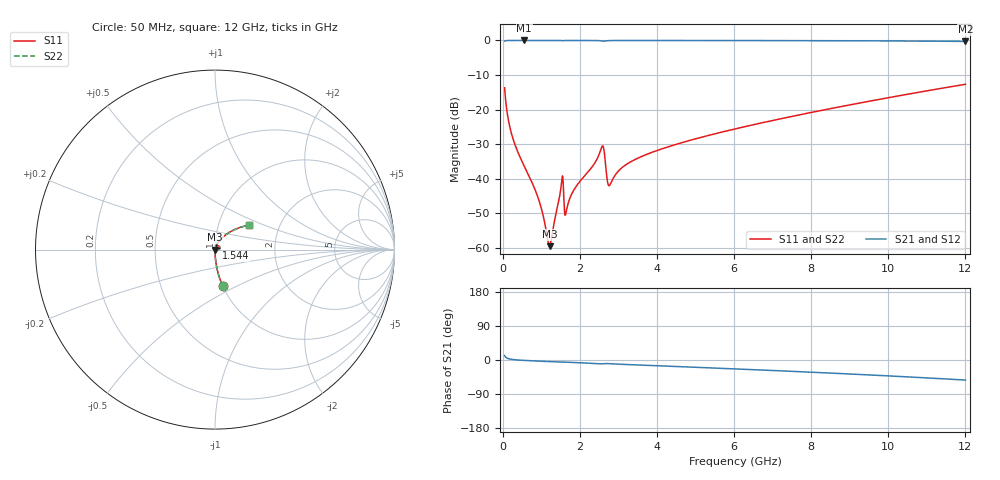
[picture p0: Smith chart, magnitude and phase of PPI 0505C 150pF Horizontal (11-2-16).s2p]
# MHz S MA R 50
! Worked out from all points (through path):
!   1601 points, 50 MHz to 12 GHz, reference 50 ohm
!   highest |S21| = -0.01 dB at 557.9 MHz (marker M1); lowest = -0.3 dB at 12 GHz (marker M2)
!   group delay of S21, straight-line fit = 12.3 ps
!   lowest |S11| = -59.5 dB at 1.215 GHz (marker M3), VSWR 1.00, Z = 50.1 - j0.00798 ohm
!   |S11| at or under -10 dB: start of sweep to end of sweep
!   |S22| runs from -59.5 to -12.7 dB; largest |S21 - S12| = 0
!   S11 on the Smith chart (normalised r, x): 50 MHz: 1.00, -0.42; 1.544 GHz: 1.02, +0.01; 12 GHz: 1.40, +0.40
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50  0.2069 -78.2  0.9781 11.8  0.9781 11.8  0.2069 -78.2
154.5625  0.06732 -86.3  0.9973 3.3  0.9973 3.3  0.06732 -86.3
236.7188  0.04311 -87.7  0.9985 1.7  0.9985 1.7  0.04311 -87.7
557.875  0.01524 -88.3  0.9991 -1.0  0.9991 -1.0  0.01524 -88.3
931.3125  0.005035 -82.5  0.999 -2.9  0.999 -2.9  0.005035 -82.5
1215.125  0.001054 -4.3  0.9989 -4.2  0.9989 -4.2  0.001054 -4.3
1274.875  0.001466 37.1  0.9988 -4.4  0.9988 -4.4  0.001466 37.1
1506.406  0.007098 62.6  0.9972 -5.6  0.9972 -5.6  0.007098 62.6
1543.75  0.01055 41.2  0.9927 -5.8  0.9927 -5.8  0.01055 41.2
1655.781  0.00349 53.9  0.9981 -5.9  0.9981 -5.9  0.00349 53.9
1805.156  0.006235 70.8  0.9985 -6.6  0.9985 -6.6  0.006235 70.8
2044.156  0.009735 73.7  0.9984 -7.6  0.9984 -7.6  0.009735 73.7
2566.969  0.02845 47.7  0.9844 -10.2  0.9844 -10.2  0.02845 47.7
2619.25  0.02754 17.4  0.9752 -9.7  0.9752 -9.7  0.02754 17.4
2716.344  0.009136 11.8  0.9913 -9.5  0.9913 -9.5  0.009136 11.8
2776.094  0.008046 42.2  0.9949 -9.9  0.9949 -9.9  0.008046 42.2
3186.875  0.01577 71.0  0.9977 -11.8  0.9977 -11.8  0.01577 71.0
4038.312  0.02594 70.5  0.9975 -15.3  0.9975 -15.3  0.02594 70.5
6025  0.05239 64.0  0.9959 -23.5  0.9959 -23.5  0.05239 64.0
8019.156  0.09113 55.9  0.9924 -32.3  0.9924 -32.3  0.09113 55.9
10013.31  0.1487 46.6  0.9846 -42.0  0.9846 -42.0  0.1487 46.6
12000  0.232 35.8  0.9672 -53.0  0.9672 -53.0  0.232 35.8
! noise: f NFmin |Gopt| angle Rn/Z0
50  0.0003787  0.861  0.3082  0.0005836
1372  0.004122  0.6832  4.708  0.002518
2701  0.01655  0.8315  9.269  0.02058
4031  0.008896  0.5948  13.59  0.003978
5360  0.011  0.5732  17.87  0.004565
6682  0.01322  0.5636  22.03  0.005269
8012  0.01557  0.5612  26.1  0.006079
9341  0.01811  0.5646  30.04  0.007029
1.067e+04  0.02092  0.5731  33.86  0.008179
1.2e+04  0.0241  0.5862  37.56  0.00961
